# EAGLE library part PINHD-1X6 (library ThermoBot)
PIN HEADER
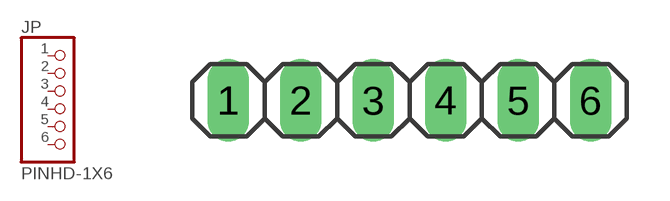
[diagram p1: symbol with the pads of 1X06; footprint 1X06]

Designator prefix JP

## PINHD-1X6TH  [1X06]
1  1  pas
2  2  pas
3  3  pas
4  4  pas
5  5  pas
6  6  pas

## Footprint 1X06 (pad centres in mm)
drill 0.95 pad 1.422 long: 1 -6.35,0; 2 -3.81,0; 3 -1.27,0; 4 1.27,0; 5 3.81,0; 6 6.35,0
